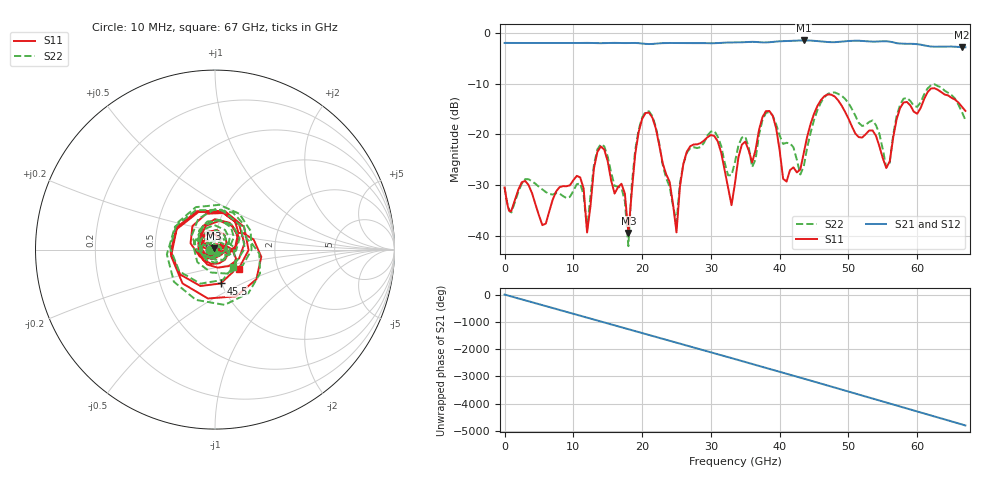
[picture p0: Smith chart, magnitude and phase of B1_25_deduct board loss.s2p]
!Keysight Technologies,N5247B,MY61255065,A.16.20.04
!Date: Sunday, September 03, 2023 21:39:23
!Correction: S11(C  2-Port  )
!S21(C  2-Port  )
!S12(C  2-Port  )
!S22(C  2-Port  )
!S2P File: Measurements: S11, S21, S12, S22:
!Deduct Board Loss
# Hz S  dB  R 50
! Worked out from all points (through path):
!   142 points, 10 MHz to 67 GHz, reference 50 ohm
!   highest |S21| = -1.45 dB at 43.5 GHz (marker M1); lowest = -2.8 dB at 66.5 GHz (marker M2)
!   lowest |S11| = -39.5 dB at 18 GHz (marker M3), VSWR 1.02, Z = 49.4 + j0.895 ohm
!   |S11| at or under -10 dB: start of sweep to end of sweep
!   |S22| runs from -42.1 to -10.1 dB; largest |S21 - S12| = 0.0023
!   S11 on the Smith chart (normalised r, x): 10 MHz: 0.94, -0.00; 45.5 GHz: 0.99, -0.39; 67 GHz: 1.27, -0.28
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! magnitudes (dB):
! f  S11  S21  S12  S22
! 10 MHz  -30.5  -1.9  -1.9  -30.5
! 11.5 GHz  -30.7  -1.9  -1.9  -32.0
! 12 GHz  -39.4  -1.9  -1.9  -38.8
! 14.5 GHz  -23.0  -2.0  -2.0  -22.4
! 18 GHz  -39.5  -2.0  -2.0  -42.1
! 20 GHz  -17.0  -2.1  -2.1  -16.7
! 22.5 GHz  -22.2  -2.0  -2.0  -21.9
! 25 GHz  -39.4  -2.0  -1.9  -37.4
! 27 GHz  -22.4  -2.0  -2.0  -22.7
! 30.5 GHz  -20.3  -2.0  -2.0  -19.3
! 33 GHz  -34.0  -1.8  -1.8  -28.1
! 34 GHz  -24.6  -1.8  -1.8  -22.2
! 36 GHz  -25.6  -1.7  -1.7  -26.5
! 38 GHz  -15.4  -1.8  -1.8  -15.8
! 40.5 GHz  -28.8  -1.6  -1.6  -21.9
! 43.5 GHz  -23.7  -1.4  -1.4  -26.3
! 45 GHz  -15.9  -1.5  -1.5  -17.1
! 45.5 GHz  -14.4  -1.6  -1.6  -15.2
! 56 GHz  -25.3  -1.7  -1.7  -25.6
! 58 GHz  -13.7  -2.1  -2.1  -13.0
! 66.5 GHz  -14.6  -2.8  -2.8  -15.6
! 67 GHz  -15.4  -2.8  -2.8  -17.2
